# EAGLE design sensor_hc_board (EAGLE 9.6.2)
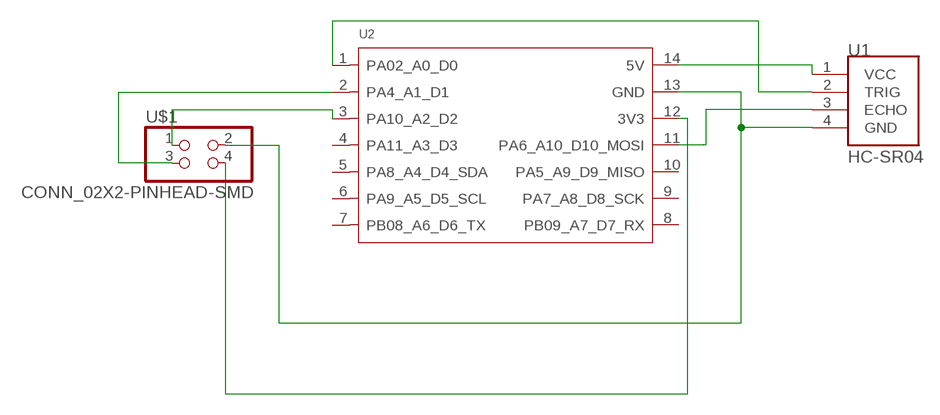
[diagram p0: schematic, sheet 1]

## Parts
U1  HC-SR04  [XCVR_HC-SR04]
U2  MOUDLE-SEEEDUINO-XIAO-SMD  [MOUDLE14P-SMD-2.54-21X17.8MM]
U$1  CONN_02X2-PINHEAD-SMD  [2X02SMD]

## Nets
N$1: U1.4(GND) U2.13(GND) U$1.2
N$2: U1.1(VCC) U2.14(5V)
N$3: U1.3(ECHO) U2.11(PA6_A10_D10_MOSI)
N$4: U1.2(TRIG) U2.1(PA02_A0_D0)
N$5: U2.3(PA10_A2_D2) U$1.1
N$6: U2.12(3V3) U$1.4
N$7: U2.2(PA4_A1_D1) U$1.3
Unconnected: U2.4(PA11_A3_D3) U2.5(PA8_A4_D4_SDA) U2.6(PA9_A5_D5_SCL) U2.7(PB08_A6_D6_TX) U2.8(PB09_A7_D7_RX) U2.9(PA7_A8_D8_SCK) U2.10(PA5_A9_D9_MISO)

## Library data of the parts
U1 = HC-SR04:HC-SR04: Ultrasonic Sensor Module Check availability; AVAILABILITY: Not in stock; DESCRIPTION: HC-SR04 Ultrasonic Sensor Qwiic Platform Evaluation Expansion Board; MF: SparkFun Electronics; MP: HC-SR04; PACKAGE: None; PRICE: None
U2 = Seeed-Studio-XIAO-RP2040-footprint-eagle:MOUDLE-SEEEDUINO-XIAO
U$1 = fab-emma-re8nowiwt7yj8fhybscymuq61o:CONN_02X2-PINHEAD-SMD

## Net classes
0 default: width 0.4 mm, clearance 0.4 mm

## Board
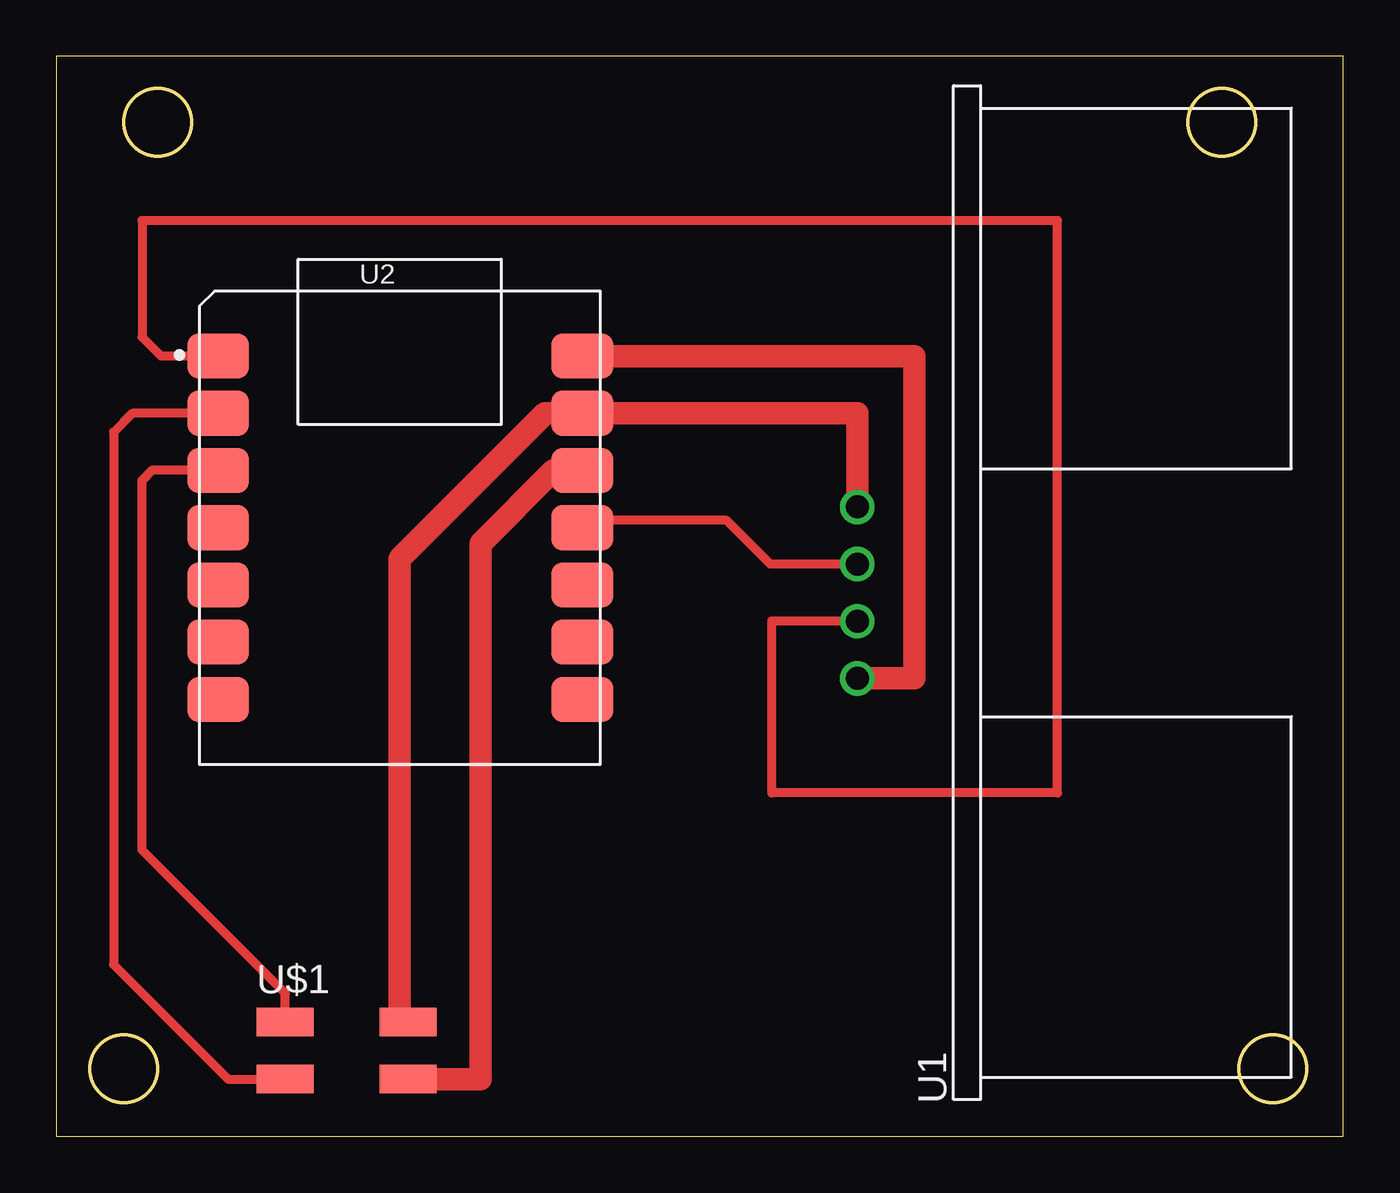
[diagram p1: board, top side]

Size 57.13 x 47.93 mm. Coordinates in mm from the lower left corner, seen from the top.
Outline: 0,0 57.13,0 57.13,47.93 0,47.93 0,0
Outline: circle at 4.5,45 radius 1.5
Outline: circle at 51.75,45 radius 1.5
Outline: circle at 3,3 radius 1.5
Outline: circle at 54,3 radius 1.5
Copper layers (1*16): Top 0.035mm / dielectric 1.5mm / Bottom 0.035mm
Design rules "default *": minimum track width 6mil, minimum drill 0.35mm, track to track 0.4mm, track to pad 0.4mm, pad to pad 0.4mm, via to via 0.4mm, smd to smd 0.4mm, copper to edge 40mil, drill to drill 6mil, minimum pad ring 10mil, minimum via ring 8mil, stop-mask expansion 4mil, vias tented up to drill 0mil, thermal gap 10mil

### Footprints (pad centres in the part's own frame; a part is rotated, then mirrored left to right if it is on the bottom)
XCVR_HC-SR04 = drill 1.02: 1 -3.81,0; 2 -1.27,0; 3 1.27,0; 4 3.81,0
MOUDLE14P-SMD-2.54-21X17.8MM = smd 2.75 x 2: 1 0.835,18.12; 2 0.835,15.58; 3 0.835,13.04; 4 0.835,10.5; 5 0.835,7.96; 6 0.835,5.42; 7 0.835,2.88; 8 17,2.88; 9 17,5.42; 10 17,7.96; 11 17,10.5; 12 17,13.04; 13 17,15.58; 14 17,18.12
2X02SMD = smd 2.54 x 1.27: 1 -2.54,1.27; 2 2.92,1.27; 3 -2.54,-1.27; 4 2.92,-1.27

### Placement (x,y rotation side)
U1  35.56,24.13 90 top
U2  6.35,16.51 0 top
U$1  12.7,3.81 0 top

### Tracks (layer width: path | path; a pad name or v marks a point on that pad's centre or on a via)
N$1
  Top 0.4: U$1.2 15.24,5.46
  Top 1: 15.24,5.46 15.24,25.64 21.69,32.09 U2.13 35.56,32.09 U1.4
N$2
  Top 1: U2.14 38.1,34.63 38.1,20.32 U1.1
N$3
  Top 0.4: U2.11 23.68,27.34 29.76,27.34 31.7,25.4 U1.3
N$4
  Top 0.4: U2.1 4.64,34.63 3.81,35.47 3.81,40.64 44.45,40.64 44.45,15.24 31.75,15.24 31.75,22.86 U1.2
N$5
  Top 0.4: U$1.1 10.16,6.35 3.81,12.7 3.81,29.11 4.25,29.55 U2.3
N$6
  Top 0.4: U2.12 22.08,29.55
  Top 1: U$1.4 18.84,2.54 18.84,26.3 22.08,29.55
N$7
  Top 0.4: U2.2 3.38,32.09 2.54,31.25 2.54,7.62 7.62,2.54 U$1.3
